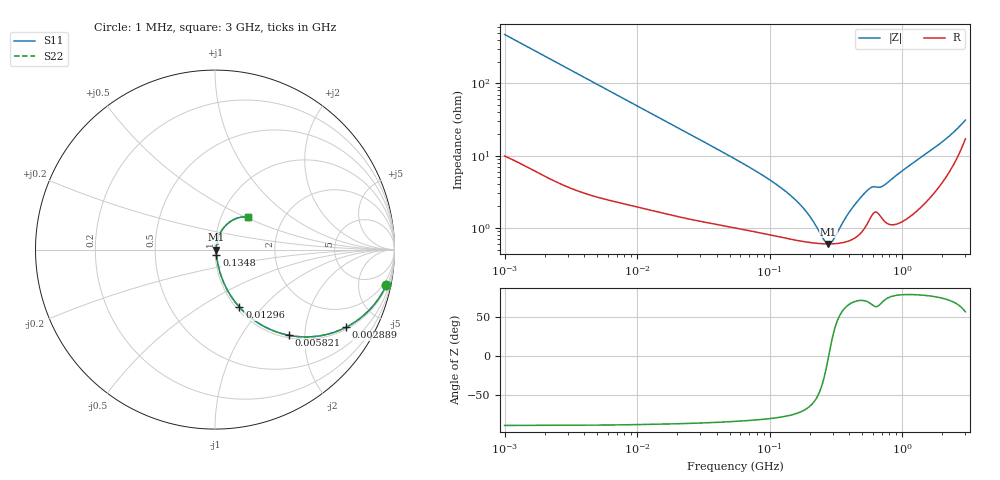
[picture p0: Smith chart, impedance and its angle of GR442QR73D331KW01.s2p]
!Murata Part Number: GR442QR73D331KW01
!These Parameters are Measured in Series Mode Connection
!Data Generated on Mar 13, 2026
!  o--ll--o
!Port1  Port2
!  o------o
!Operation Temp=25[degC], DC Bias Voltage=0[V]
!Freq. Start=1000[kHz] Stop=3[GHz] 401[Steps]
# Hz S RI R 50
!Freq.(Hz) S11(Real) S11(Imag) S21(Real) S21(Imag) S12(Real) S12(Imag) S22(Real) S22(Imag)
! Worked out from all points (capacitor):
!   401 points, 1 MHz to 3 GHz, reference 50 ohm
!   read as one part in series: C = 334 pF near 1.041 MHz
!   lowest |Z| = 602 mohm at 277.1 MHz (marker M1)
!   series resonance near 278.8 MHz, so ESL is about 980 pH
!   S11 on the Smith chart (normalised r, x): 1 MHz: 1.20, -9.49; 2.889 MHz: 1.08, -3.33; 5.821 MHz: 1.05, -1.66; 12.96 MHz: 1.03, -0.75; 134.8 MHz: 1.01, -0.06; 3 GHz: 1.34, +0.52
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1000000  0.9537 -0.1999  0.0463 0.1999  0.0463 0.1999  0.9537 -0.1999
1751453  0.8767 -0.3181  0.1233 0.3181  0.1233 0.3181  0.8767 -0.3181
2888807  0.7305 -0.4325  0.2695 0.4325  0.2695 0.4325  0.7305 -0.4325
3823119  0.6116 -0.4752  0.3884 0.4752  0.3884 0.4752  0.6116 -0.4752
5820586  0.4117 -0.4775  0.5883 0.4775  0.5883 0.4775  0.4117 -0.4775
8686058  0.247 -0.4131  0.753 0.4131  0.753 0.4131  0.247 -0.4131
1.29622e7  0.1361 -0.3205  0.8639 0.3205  0.8639 0.3205  0.1361 -0.3205
1.461624e7  0.1128 -0.2927  0.8872 0.2927  0.8872 0.2927  0.1128 -0.2927
5.477226e7  0.0176 -0.087  0.9824 0.087  0.9824 0.087  0.0176 -0.087
1.348146e8  0.00799 -0.0298  0.992 0.0298  0.992 0.0298  0.00799 -0.0298
1.714156e8  0.00692 -0.0194  0.9931 0.0194  0.9931 0.0194  0.00692 -0.0194
2.094008e8  0.00632 -0.0112  0.9937 0.0112  0.9937 0.0112  0.00632 -0.0112
2.558035e8  0.00601 -0.00338  0.994 0.00338  0.994 0.00338  0.00601 -0.00338
2.771263e8  0.00598 -0.000233  0.994 0.000233  0.994 0.000233  0.00598 -0.000233
3.002264e8  0.00601 0.00295  0.994 -0.00295  0.994 -0.00295  0.00601 0.00295
3.973271e8  0.00681 0.0148  0.9932 -0.0148  0.9932 -0.0148  0.00681 0.0148
5.258324e8  0.0109 0.0285  0.9891 -0.0285  0.9891 -0.0285  0.0109 0.0285
5.81181e8  0.015 0.0323  0.985 -0.0323  0.985 -0.0323  0.015 0.0323
6.958997e8  0.0149 0.0334  0.9851 -0.0334  0.9851 -0.0334  0.0149 0.0334
8.005644e8  0.0129 0.0421  0.9871 -0.0421  0.9871 -0.0421  0.0129 0.0421
1.931433e9  0.0548 0.1292  0.9452 -0.1292  0.9452 -0.1292  0.0548 0.1292
3e9  0.1858 0.1806  0.8142 -0.1806  0.8142 -0.1806  0.1858 0.1806
